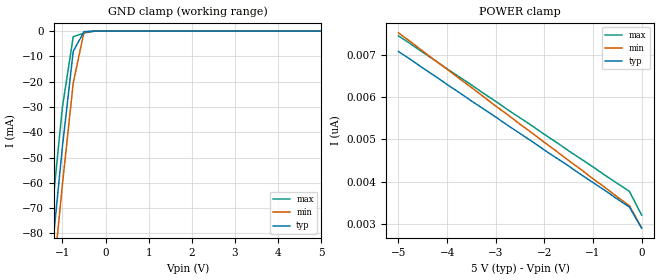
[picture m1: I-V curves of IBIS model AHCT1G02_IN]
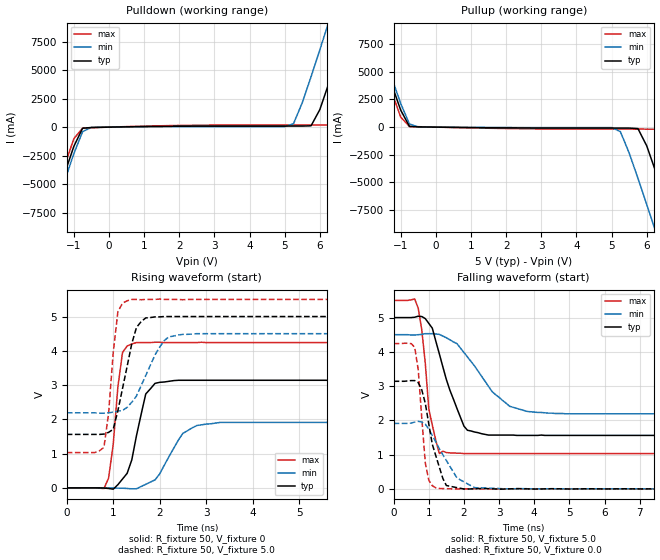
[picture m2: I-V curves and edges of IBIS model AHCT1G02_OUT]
| TEXAS INSTRUMENTS INCORPORATED
| Standard Linear and Logic Group
| IBIS Model of SN74AHCT1G02
| SINGLE 2-INPUT POSITIVE-NOR GATE
| SOT 5-pin (DCK) and SOT 5-pin (DBV) Package
[IBIS Ver]   3.2
[Comment Char]  |_char
[File Name]   ahct1g02.ibs
[File Rev]   2.0 J_die
[Date]   May 24, 2000
[Source]   Data created from HSPICE simulations at TI-SLL.
[Notes]   The following is an IBIS list for the AHCT1G02.
|   Please contact sllibis@ti.com with questions and
|   comments concerning SLL IBIS models.
[Disclaimer] Property of Texas Instruments Incorporated.  Unauthorized
   reproduction and/or distribution is strictly prohibited.
   This product is protected under copyright law.
   Created 2000, (C) Copyright 2000, Texas Instruments Inc.,
   All Rights Reserved.
   UNLESS THERE IS A SIGNED, WRITTEN AGREEMENT TO THE
   CONTRARY, TEXAS INSTRUMENTS () IS PROVIDING THE IBIS
   MODELS  AND WITHOUT ANY WARRANTY, EXPRESSED OR
   IMPLIED.  TI assumes no liability for:
   1) the accuracy of the IBIS models provided to your
   company;
   2) the proper functioning of these IBIS Models in your
   design or for any resulting applications; or
   3) infringement of patents, copyrights or intellectual
   property rights resulting from your use of these IBIS
   models.
   TI provides IBIS Models as a service to our customers.
   You and your company shall not distribute, sell or give
   these models to anyone else without prior written
   permission from TI.
   TI reserves the right to make changes to our products or
   to discontinue any semiconductor product or service
   without notice, and advises our customers to obtain the
   latest version of relevant information to verify, before
   placing orders, that the information being relied on is
   current.
   Please be aware that your receipt and use of the IBIS
   information provided shall serve as acceptance of these
   terms and conditions.  If you do not accept these terms,
   you should return or destroy the IBIS models and any
   other accompanying information immediately.
|   Component AHCT1G02_DCK
[Component]   AHCT1G02_DCK
[Manufacturer]  Texas Instruments, Inc.
[Package]
|   typ   min   max
R_pkg   0.020   0.017   0.025
L_pkg   0.998nH   0.881nH   1.069nH
C_pkg   0.146pF   0.118pF   0.205pF
[Pin]   signal_name   model_name   R_pin   L_pin   C_pin
1   A   AHCT1G02_IN   0.019   1.069nH   0.162pF
2   B   AHCT1G02_IN   0.018   0.881nH   0.121pF
3   GND   GND   0.017   1.031nH   0.205pF
4   Y   AHCT1G02_OUT   0.020   0.960nH   0.124pF
5   VCC   POWER   0.025   1.049nH   0.118pF
|   Component AHCT1G02_DBV
[Component]   AHCT1G02_DBV
[Manufacturer]  Texas Instruments, Inc.
[Package]
|   typ   min   max
R_pkg   0.025   0.021   0.029
L_pkg   1.529nH   1.312nH   1.906nH
C_pkg   0.156pF   0.110pF   0.240pF
[Pin]   signal_name   model_name   R_pin   L_pin   C_pin
1   A   AHCT1G02_IN   0.021   1.511nH   0.144pF
2   B   AHCT1G02_IN   0.023   1.312nH   0.138pF
3   GND   GND   0.029   1.906nH   0.240pF
4   Y   AHCT1G02_OUT   0.026   1.541nH   0.150pF
5   VCC   POWER   0.025   1.374nH   0.110pF
| Models and submodels in the file (2): AHCT1G02_IN (Input), AHCT1G02_OUT (Output)
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|   Model AHCT1G02_IN
[Model]   AHCT1G02_IN
Model_type  Input
Polarity   Inverting
Vinl = 0.8
Vinh = 2.0
| variable   typ   min   max
C_comp   1.24pf   0.93pf   1.55pf
[Temperature Range]   25   85   -40
[Voltage Range]   5.0   4.5   5.5
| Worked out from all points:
|   GND clamp passes 1 mA (typ) near -0.52 V on its own axis
[GND Clamp]
|   Voltage   I(typ)   I(min)   I(max)
-5V       -773mA     -786mA     -758mA
-1.5V     -133mA     -148mA     -117mA
-1.25V    -88.7mA    -104mA     -72.7mA
-1V       -45.6mA    -60.5mA    -30mA
-750mV    -7.99mA    -20.5mA    -2.23mA
-500mV    -233uA     -353uA     -759uA
-250mV    -2.63nA    -182nA     -26.9uA
5V        2.9nA      3.64nA     2.54nA
[POWER Clamp]
|   Voltage   I(typ)   I(min)   I(max)
-5V       7.08nA     7.52nA     7.45nA
-1.5V     4.37nA     4.5nA      4.73nA
-250mV    3.4nA      3.43nA     3.77nA
0V        2.9nA      2.91nA     3.21nA
|   Model AHCT1G02_OUT
[Model]   AHCT1G02_OUT
Model_type  Output
Polarity   Inverting
Vmeas = 2.50v
Cref = 15pf
| variable   typ   min   max
C_comp   3.12pf   2.34pf   3.90pf
[Temperature Range]   25   85   -40
[Voltage Range]   5.0   4.5   5.5
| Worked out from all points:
|   slope of the pulldown table from 0 to 0.75 V, typ, clamps not added: 18.8 ohm
|   slope of the pullup table from 0 to 0.75 V, typ, clamps not added: 25.3 ohm
|   rising waveform, R_fixture 50, V_fixture 0: 20-80 % time 310ps typ, 484ps min, 187ps max; typ from 0 V to 3.14 V
|   falling waveform, R_fixture 50, V_fixture 5.0: 20-80 % time 640ps typ, 1.06ns min, 283ps max; typ from 5 V to 1.56 V
|   rising waveform, R_fixture 50, V_fixture 5.0: 20-80 % time 322ps typ, 484ps min, 180ps max; typ from 1.56 V to 5 V
|   falling waveform, R_fixture 50, V_fixture 0.0: 20-80 % time 405ps typ, 647ps min, 188ps max; typ from 3.14 V to 0 V
[Pulldown]
|   Voltage   I(typ)   I(min)   I(max)
-5V       -40.9A     -41.4A     -40.3A
-1.75V    -8.76A     -9.39A     -8.09A
-1V       -1.69A     -2.33A     -1.02A
-750mV    -95.5mA    -395mA     -80.6mA
5.25V     93.4mA     298mA      192mA
5.75V     116mA      4.42A      192mA
6.25V     3.8A       9.19A      193mA
6.5V      6.17A      11.6A      931mA
6.75V     8.59A      14.1A      3.15A
7.25V     13.5A      19A        7.96A
7.5V      15.9A      21.4A      10.4A
10V       40.7A      46.2A      35.2A
[Pullup]
|   Voltage   I(typ)   I(min)   I(max)
-5V       40.7A      41.2A      40.1A
-2V       11A        11.6A      10.4A
-1.75V    8.59A      9.19A      7.96A
-1V       1.54A      2.14A      907mA
-750mV    63.6mA     284mA      62.5mA
5.25V     -84.4mA    -401mA     -178mA
5.75V     -130mA     -4.62A     -178mA
6.25V     -3.97A     -9.39A     -187mA
6.75V     -8.76A     -14.3A     -3.28A
7.25V     -13.6A     -19.2A     -8.09A
7.5V      -16.1A     -21.6A     -10.5A
10V       -40.9A     -46.4A     -35.3A
[Ramp]
| variable   typ   min   max
dV/dt_r   1.91E+00/3.51E-10   1.19E+00/5.51E-10   2.55E+00/1.46E-10
dV/dt_f   2.09E+00/5.55E-10   1.41E+00/1.03E-09   2.72E+00/2.74E-10
R_load = 50
[Rising Waveform]
R_fixture = 50
V_fixture = 0
|   Time   V(typ)   V(min)   V(max)
0s        0V         0V         0V
800ps     -5.25mV    1mV        -19.1mV
1ns       -37.7mV    -3.6mV     1.27V
1.2ns     259mV      -9.88mV    3.95V
1.5ns     1.52V      -25.5mV    4.24V
1.7ns     2.74V      104mV      4.24V
1.9ns     3.05V      233mV      4.25V
2.5ns     3.14V      1.59V      4.24V
3.3ns     3.14V      1.91V      4.24V
25ns      3.14V      1.91V      4.24V
[Falling Waveform]
R_fixture = 50
V_fixture = 5.0
V_fixture_min = 4.5
V_fixture_max = 5.5
|   Time   V(typ)   V(min)   V(max)
0s        5V         4.5V       5.5V
700ps     5.04V      4.5V       5.27V
900ps     4.97V      4.53V      3.67V
1ns       4.83V      4.53V      2.33V
1.3ns     3.94V      4.51V      1.03V
2ns       1.83V      3.98V      1.03V
2.7ns     1.57V      2.99V      1.03V
3.3ns     1.57V      2.41V      1.03V
4.6ns     1.56V      2.2V       1.03V
25ns      1.56V      2.19V      1.03V
[Rising Waveform]
R_fixture = 50
V_fixture = 5.0
V_fixture_min = 4.5
V_fixture_max = 5.5
|   Time   V(typ)   V(min)   V(max)
0s        1.56V      2.19V      1.03V
800ps     1.57V      2.18V      1.18V
900ps     1.62V      2.19V      2.17V
1ns       1.71V      2.21V      3.95V
1.1ns     2.25V      2.24V      5.14V
1.4ns     4.21V      2.5V       5.5V
1.6ns     4.85V      2.98V      5.49V
2.1ns     5V         4.3V       5.5V
2.5ns     5V         4.48V      5.49V
25ns      5V         4.5V       5.5V
[Falling Waveform]
R_fixture = 50
V_fixture = 0.0
|   Time   V(typ)   V(min)   V(max)
0s        3.14V      1.91V      4.24V
600ps     3.16V      1.95V      4.13V
700ps     3.1V       1.97V      3.47V
900ps     2.5V       1.89V      762mV
1ns       1.89V      1.74V      253mV
1.3ns     633mV      1.17V      11.3mV
1.5ns     97.3mV     827mV      5.1mV
1.8ns     36.1mV     321mV      -966uV
2.3ns     3.32mV     35.4mV     1.16mV
25ns      0V         0V         0V
